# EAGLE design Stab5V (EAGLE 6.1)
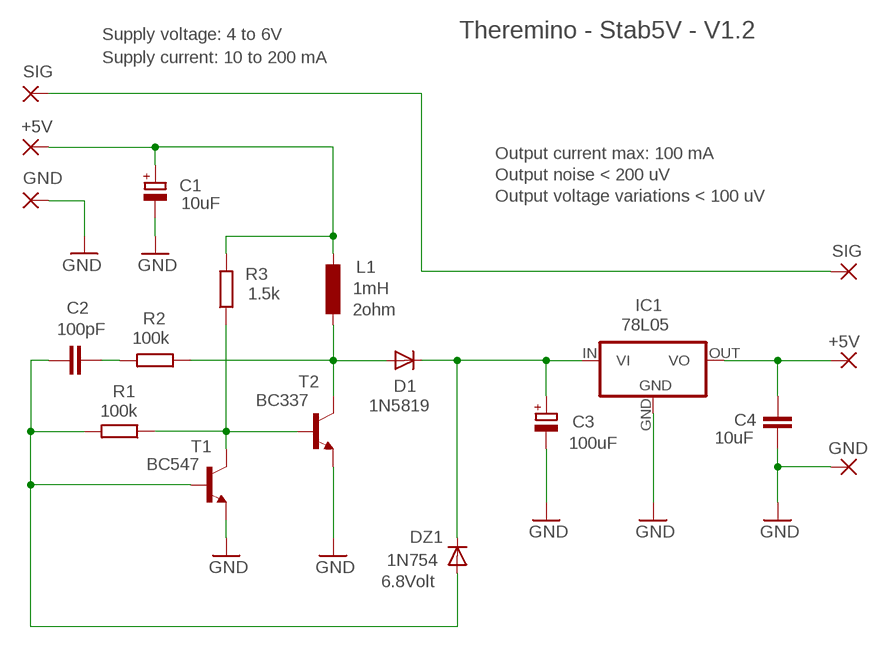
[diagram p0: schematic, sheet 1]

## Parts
C1  10uF  CPOL-EUE2-5B  [E2-5B]
C2  100pF  C-EU025-024X044  [C025-024X044]
C3  100uF  CPOL-EUTT2D4L  [TT2D4L]
C4  10uF  C-EUC0805  [C0805]
D1  1N5819  DIODE-DO34-7  [DO34-7]
DZ1  1N754  DIODE-DO34-7  [DO34-7]
IC1  78L05  78REG  [TO92-REG]
L1  1mH  INDUCTORL_VERT_508  [L_VERT_508]
PAD1  GND  WIREPAD1,6/0,8  [1,6/0,8]
PAD2  +5V  WIREPAD1,6/0,8  [1,6/0,8]
PAD3  SIG  WIREPAD1,6/0,8  [1,6/0,8]
PAD4  GND  WIREPAD1,6/0,8  [1,6/0,8]
PAD5  +5V  WIREPAD1,6/0,8  [1,6/0,8]
PAD6  SIG  WIREPAD1,6/0,8  [1,6/0,8]
R1  100k  R-EU_0204/5  [0204/5]
R2  100k  R-EU_0204/5  [0204/5]
R3  1.5k  R-EU_0204/5  [0204/5]
T1  BC547  -NPN-TO92-CBE  [TO92-CBE]
T2  BC337  -NPN-TO92-CBE  [TO92-CBE]

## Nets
+5V: C1.+ L1.+ PAD2.1(P) R3.2
GND: C1.- C3.- C4.2 IC1.GND PAD1.1(P) PAD4.1(P) T1.E T2.E
N$1: C3.+ D1.C DZ1.C IC1.IN(VI)
N$2: C2.2 R2.2
N$3: PAD3.1(P) PAD6.1(P)
N$4: C2.1 DZ1.A R1.2 T1.B
N$6: D1.A L1.- R2.1 T2.C
N$15: C4.1 IC1.OUT(VO) PAD5.1(P)
N$26: R1.1 R3.1 T1.C T2.B

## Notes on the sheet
- Supply voltage: 4 to 6V | Theremino - Stab5V - V1.2
- Supply current: 10 to 200 mA
- Output current max: 100 mA
- Output noise < 200 uV
- Output voltage variations < 100 uV

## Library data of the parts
C1 C3 = 00-LIVIO:CPOL-EU: POLARIZED CAPACITOR, European symbol
C2 C4 = 00-LIVIO:C-EU: CAPACITOR, European symbol
D1 = 00-LIVIO:DIODE-: DIODE
DZ1 = 00-LIVIO:DIODE-: DIODE; VOLTAGE: 6.8Volt
IC1 = 00-LIVIO:78*: Positive VOLTAGE REGULATOR Source: http://cache.national.com/ds/LM/LM78L05.pdf http://www.fairchildsemi.com/ds/LM/LM7805.pdf
L1 = 00-LIVIO:INDUCTOR; RES: 2ohm
PAD1-PAD6 = 00-LIVIO:WIREPAD: Wire PAD connect wire on PCB
R1-R3 = 00-LIVIO:R-EU_: RESISTOR, European symbol
T1 T2 = 00-LIVIO:*-NPN-: NPN Transistror

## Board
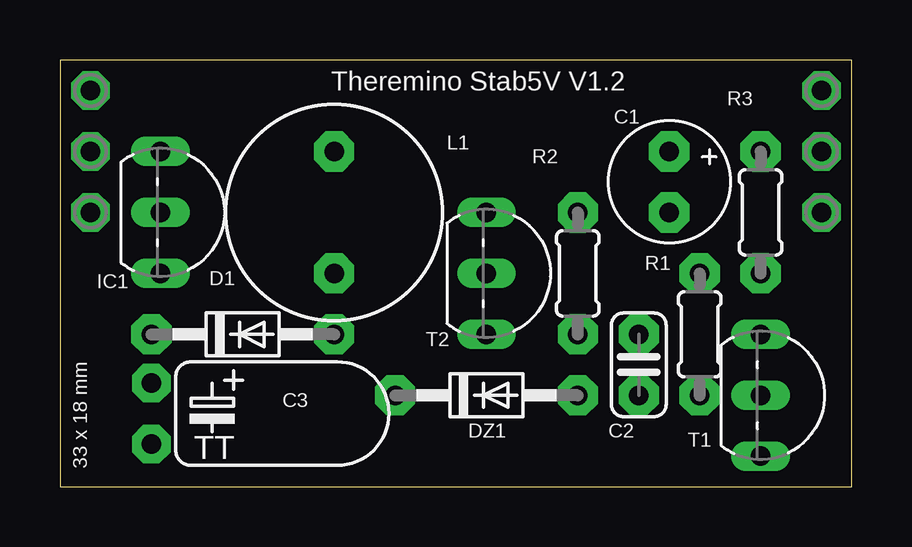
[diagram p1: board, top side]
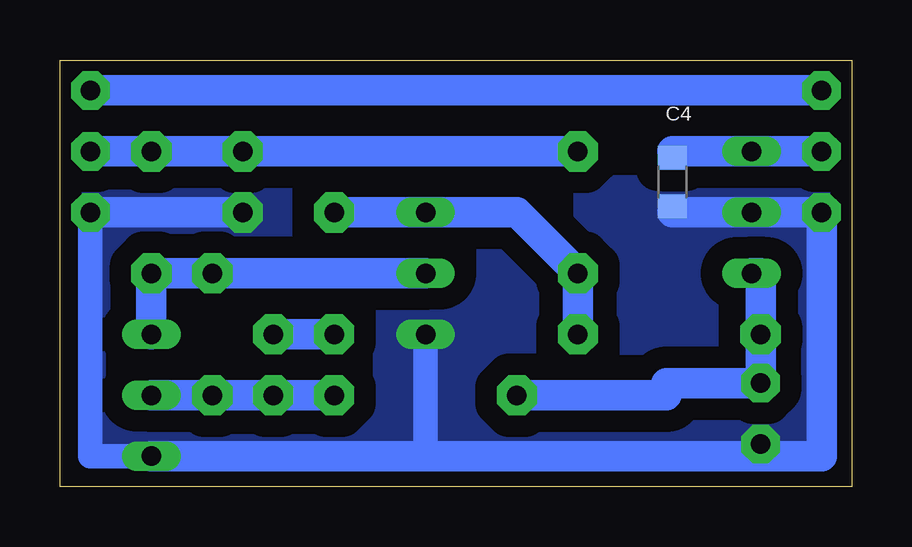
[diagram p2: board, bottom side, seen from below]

Size 33.02 x 17.78 mm. Coordinates in mm from the lower left corner, seen from the top.
Outline: 0,0 33.02,0 33.02,17.78 0,17.78 0,0
Copper layers (1*16): Top 0.035mm / dielectric 1.5mm / Bottom 0.035mm
Design rules: minimum track width 10mil, minimum drill 0.6mm, track to track 8mil, track to pad 8mil, pad to pad 8mil, via to via 8mil, smd to smd 8mil, copper to edge 31mil, drill to drill 8mil, minimum pad ring 5mil, minimum via ring 8mil, stop-mask expansion 4mil, vias tented up to drill 0mil, thermal gap 47mil
bRestrict: 2 lines

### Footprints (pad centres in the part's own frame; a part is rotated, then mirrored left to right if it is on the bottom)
E2-5B = drill 0.813 pad 1.676 octagon: + -1.27,0; - 1.27,0
C025-024X044 = drill 0.813 pad 1.676 octagon: 1 -1.27,0; 2 1.27,0
TT2D4L = drill 0.813 pad 1.6 octagon: + -1.27,0; - 1.27,0
C0805 = smd 1 x 1.2: 1 -1.016,0; 2 1.016,0
DO34-7 = drill 0.813 pad 1.676 octagon: A 3.81,0; C -3.81,0
TO92-REG = drill 0.813 long: GND 0,0; IN 2.54,0; OUT -2.54,0
L_VERT_508 = drill 0.813 pad 1.676 octagon: + -2.54,0; - 2.54,0
1,6/0,8 = drill 0.813 pad 1.6 octagon: 1 0,0
0204/5 = drill 0.813 pad 1.676 octagon: 1 -2.54,0; 2 2.54,0
TO92-CBE = drill 0.813 long: B 0,0; C -2.54,0; E 2.54,0

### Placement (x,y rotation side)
C1  25.4,12.7 270 top
C2  24.13,5.08 90 top
C3  3.81,3.05 270 top
C4  7.49,12.7 270 bottom
D1  7.62,6.35 0 top
DZ1  17.78,3.81 0 top
IC1  4.19,11.43 270 top
L1  11.43,11.43 270 top
PAD1  31.75,11.43 0 top
PAD2  31.75,13.97 0 top
PAD3  31.75,16.51 0 top
PAD4  1.27,11.43 0 top
PAD5  1.27,13.97 0 top
PAD6  1.27,16.51 0 top
R1  26.67,6.35 270 top
R2  21.59,8.89 270 top
R3  29.21,11.43 90 top
T1  29.21,3.81 270 top
T2  17.78,8.89 270 top

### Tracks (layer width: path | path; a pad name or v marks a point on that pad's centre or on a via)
+5V
  Bottom 1.27: L1.+ C1.+ R3.2 PAD2.1
GND
  Bottom 1.016: T2.E 17.78,1.27 | PAD1.1 31.75,1.27 T1.E | 7.49,11.43 C4.2
  Bottom 1.27: 3.81,1.27 1.27,1.27 PAD4.1 IC1.GND 7.49,11.43 | 3.81,1.27 17.78,1.27 T1.E | C3.- 3.81,1.27 | C1.- PAD1.1
  pour Bottom (isolate 0.9, rank 6, no thermals): -1,-1 34.02,-1 34.02,18.78 -1,18.78
N$1
  Bottom 1.27: IC1.IN 3.81,8.89 D1.C C3.+ 7.75,4.32 7.75,3.81 DZ1.C
N$2
  Bottom 1.27: R2.2 C2.2
N$3
  Bottom 1.27: PAD6.1 PAD3.1
N$4
  Bottom 1.016: C2.1 T1.B
  Bottom 1.27: T1.B R1.2 C2.1 DZ1.A
N$6
  Bottom 1.27: R2.1 T2.C 13.97,11.43 L1.- D1.A
N$15
  Bottom 1.016: 7.49,13.97 C4.1
  Bottom 1.27: PAD5.1 IC1.OUT 7.49,13.97
N$26
  Bottom 1.27: T1.C R3.1 R1.1 T2.B

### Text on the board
tNames: Theremino Stab5V V1.2 | 33 x 18 mm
